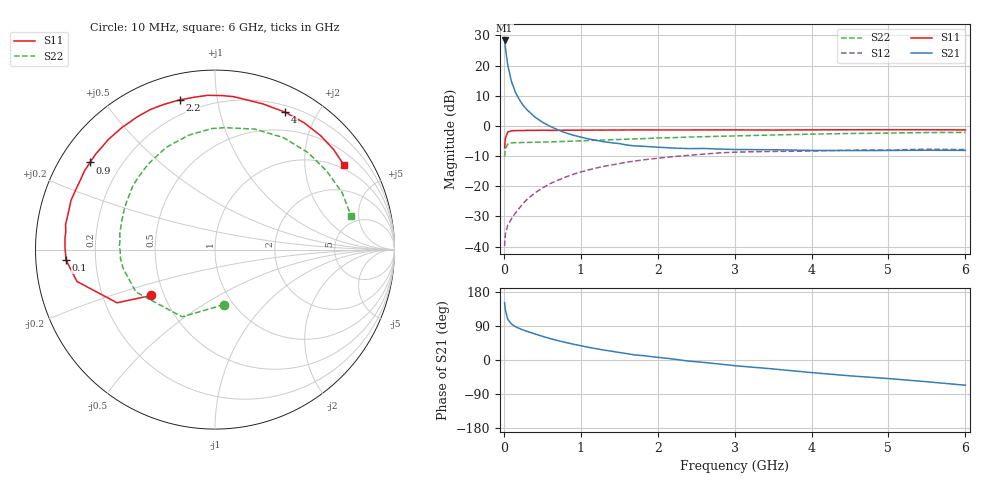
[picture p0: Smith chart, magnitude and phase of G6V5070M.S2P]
! SIEMENS Small Signal Semiconductors
! BFG193
! Si NPN RF Bipolar Junction Transistor in SOT223
! VCE = 0.5 V  IC = 70 mA
! Common Emitter S-Parameters:  August  1996
# GHz  S  MA  R  50
!  f  S11  S21  S12  S22
! GHz  MAG  ANG  MAG  ANG  MAG  ANG  MAG  ANG
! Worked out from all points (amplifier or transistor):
!   36 points, 10 MHz to 6 GHz, reference 50 ohm
!   highest |S21| = 28.3 dB at 10 MHz (marker M1)
!   |S21| within 3 dB of that: start of sweep to 23.69 MHz
!   unconditionally stable (mu >= 1): start of sweep to 18.78 MHz; 87.72 MHz to end of sweep
!   at 250 MHz: K = 1.37, MAG = 12.7 dB, |S12| = -25.7 dB
!   at 1.4 GHz: K = 1.27, MAG = 0.6 dB, |S12| = -13.0 dB
!   at 6 GHz: K = 1.07, MAG = -1.8 dB, |S12| = -7.8 dB
!   S11 on the Smith chart (normalised r, x): 10 MHz: 0.43, -0.27; 100 MHz: 0.09, -0.03; 900 MHz: 0.09, +0.31; 2.2 GHz: 0.12, +0.78; 4 GHz: 0.27, +1.60; 6 GHz: 0.87, +3.12
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0.01  0.4367 -144.2  26 151.2  0.0102 57.4  0.311 -80.8
0.02  0.621 -151.5  19.97 132.3  0.0161 47.9  0.4169 -116.1
0.05  0.7893 -167.0  10.29 107.6  0.0226 40.6  0.4999 -151.8
0.1  0.8318 -176.0  5.395 94.9  0.0291 46.9  0.522 -168.2
0.15  0.8359 179.0  3.632 87.9  0.0361 52.5  0.5291 -174.7
0.2  0.838 175.7  2.746 83.2  0.0434 56.9  0.5282 -178.8
0.25  0.8374 173.1  2.205 79.2  0.052 59.1  0.5328 177.7
0.3  0.8442 170.5  1.856 75.7  0.0604 60.4  0.5316 175.3
0.4  0.8426 165.5  1.416 69.0  0.0768 61.2  0.5375 170.4
0.5  0.8478 161.2  1.155 62.6  0.0935 60.1  0.54 166.2
0.6  0.8447 157.0  0.986 56.7  0.1104 58.8  0.5437 162.5
0.7  0.8444 152.8  0.864 51.4  0.1258 56.8  0.5482 158.9
0.9  0.8486 145.1  0.704 41.9  0.1581 52.1  0.5598 151.4
1.1  0.8504 137.9  0.609 33.5  0.1866 47.1  0.5725 144.8
1.7  0.8577 117.5  0.466 13.5  0.2616 30.7  0.6094 124.8
2.2  0.8572 103.2  0.43 2.6  0.3099 16.4  0.6388 109.3
2.8  0.8592 87.3  0.414 -10.6  0.357 0.5  0.6749 91.3
3.5  0.8545 71.8  0.403 -23.6  0.3778 -17.8  0.7074 71.6
4  0.8597 62.9  0.393 -33.2  0.3835 -27.1  0.7314 58.5
4.5  0.8635 54.8  0.39 -41.8  0.3968 -36.3  0.7487 46.2
5.5  0.8647 40.3  0.395 -57.4  0.4126 -56.8  0.7763 24.1
6  0.859 33.3  0.393 -66.6  0.4054 -68.4  0.7808 13.8
